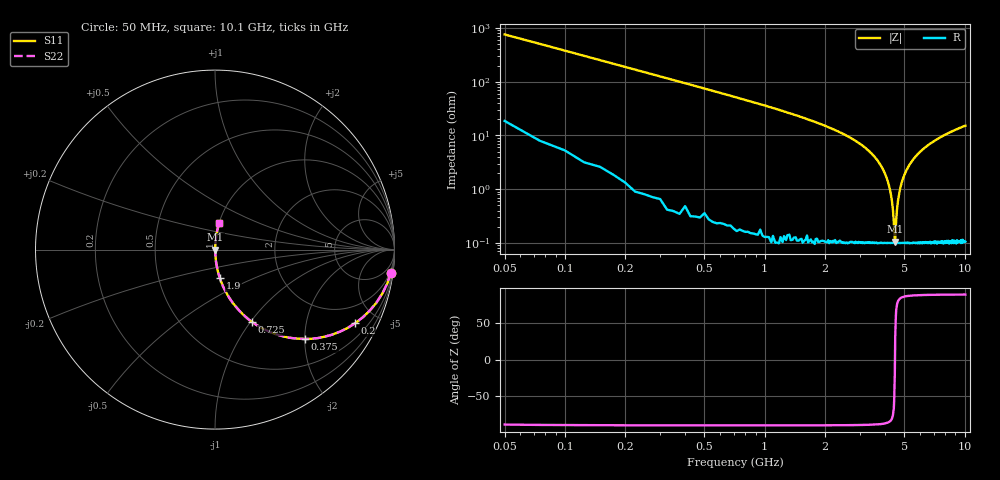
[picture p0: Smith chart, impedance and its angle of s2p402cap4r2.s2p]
! AVX Thin Film Operation		Date: April 2003
! Description: Accu-P® Series, Thin Film, SMD, RF Capacitor
! Part Number: 04025J4R2ABS
! 50 MHz  -  10.05 GHz
! Serial Measurements
# hz S db R 50
!	S11		S21		S12		S22
!	dB	Phase	dB	Phase	dB	Phase	dB	Phase
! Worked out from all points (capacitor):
!   400 points, 50 MHz to 10.1 GHz, reference 50 ohm
!   read as one part in series: C = 4.2 pF near 100 MHz
!   lowest |Z| = 105 mohm at 4.48 GHz (marker M1)
!   series resonance near 4.487 GHz, so ESL is about 300 pH
!   S11 on the Smith chart (normalised r, x): 50 MHz: 1, -15; 200 MHz: 1.03, -3.78; 375 MHz: 1.01, -2.01; 725 MHz: 1.00, -1.02; 1.9 GHz: 1.00, -0.33; 10.1 GHz: 1.00, +0.30
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5e7  -0.10 -7.5  -17.70 81.1  -17.70 81.1  -0.10 -7.5
1e8  -0.32 -14.7  -11.90 74.5  -11.90 74.5  -0.32 -14.7
2e8  -1.10 -27.8  -6.63 61.8  -6.63 61.8  -1.10 -27.8
3.75e8  -3.01 -44.8  -3.04 45.0  -3.04 45.0  -3.01 -44.8
7.25e8  -6.88 -62.9  -1.01 26.9  -1.01 26.9  -6.88 -62.9
1.73e9  -14.70 -79.1  -0.16 10.6  -0.16 10.6  -14.70 -79.1
1.9e9  -15.80 -80.3  -0.12 9.3  -0.12 9.3  -15.80 -80.3
3.4e9  -26.50 -86.1  -0.02 2.7  -0.02 2.7  -26.50 -86.1
3.88e9  -32.10 -86.3  -0.01 1.4  -0.01 1.4  -32.10 -86.3
4.18e9  -38.30 -84.6  -0.01 0.7  -0.01 0.7  -38.30 -84.6
4.38e9  -47.40 -76.2  -0.01 0.2  -0.01 0.2  -47.40 -76.2
4.43e9  -52.30 -65.7  -0.01 0.1  -0.01 0.1  -52.30 -65.7
4.48e9  -59.60 -18.1  -0.01 0.0  -0.01 0.0  -59.60 -18.1
4.5e9  -58.60 31.5  -0.01 -0.0  -0.01 -0.0  -58.60 31.5
4.6e9  -47.10 76.7  -0.01 -0.2  -0.01 -0.2  -47.10 76.7
4.7e9  -41.90 82.4  -0.01 -0.5  -0.01 -0.5  -41.90 82.4
4.85e9  -37.50 84.9  -0.01 -0.8  -0.01 -0.8  -37.50 84.9
5.08e9  -33.60 86.1  -0.01 -1.2  -0.01 -1.2  -33.60 86.1
5.8e9  -27.10 86.2  -0.02 -2.5  -0.02 -2.5  -27.10 86.2
6.75e9  -23.00 85.1  -0.03 -4.1  -0.03 -4.1  -23.00 85.1
8.43e9  -18.90 83.0  -0.06 -6.5  -0.06 -6.5  -18.90 83.0
1.01e10  -16.50 81.0  -0.11 -8.6  -0.11 -8.6  -16.50 81.0
